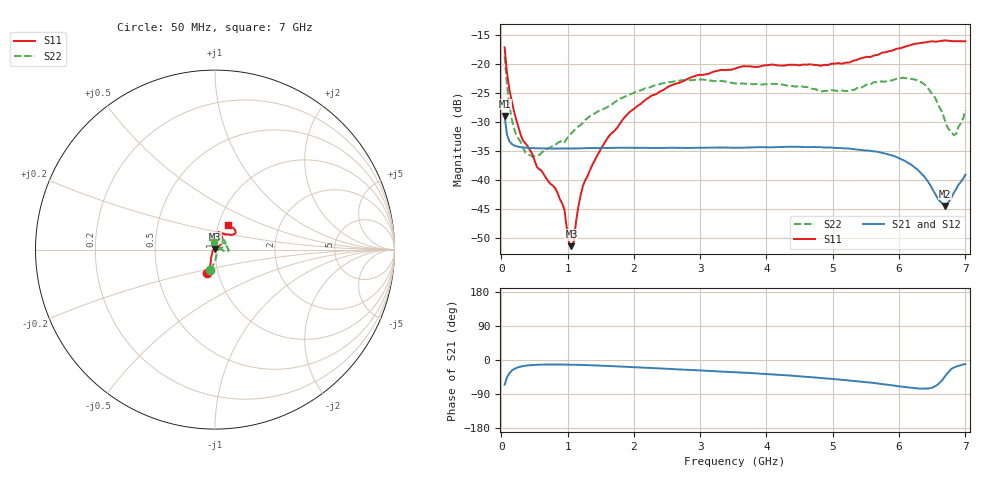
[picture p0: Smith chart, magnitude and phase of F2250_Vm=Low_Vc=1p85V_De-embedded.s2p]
! Integrated Device Technology
! Corporate Headquarters
! 6024 Silver Creek Valley Road
! San Jose, CA 95138  USA
! Phone:  1-408-284-8200
! Toll Free:  1-800-223-1366
! Webpage:  http://www.idt.com/
! Timing and RF Division
! 515 Groton Road, Suite 102
! Westford, MA 01886-6024
! Device:  F2250
! Description: Voltage Variable RF Attenuator
! Frequency:  50.0 -  6000.00 MHz
! Package:  3x3 mm Thin QFN Plastic Package: 16 pin
! Ports:  2 RF, 3 DC
!  Pin  1  = GND
!  Pin  2  = NC
!  Pin  3  = RF1  = Port 1
!  Pin  4  = NC
!  Pin  5  = GND
!  Pin  6  = GND
!  Pin  7  = GND
!  Pin  8  = GND
!  Pin  9  = NC
!  Pin 10  = RF2  = Port 2
!  Pin 11  = NC
!  Pin 12  = GND
!  Pin 13  = GND
!  Pin 14  = VCNTRL
!  Pin 15  = VDD
!  Pin 16  = VMODE
! Vcntrl:  1.850 Volts
! Vmode:  +0.000 Volts
! Vdd:  +3.30  Volts
! Current:  1.186 mA
! Data:  The device was measured on a the F2250 evaluation board which has
!  individual transmission lines to the RF pins.  Data was collected
!  using a calibrated network analyzer.  The evaluation board was
!  de-embedded using a TRL calibration technique.
!  The reference plane is the edge of the package pin.
! Misc:  SN 10
!  Action Tracker AT0258
! Date Measured:  2014-11-26
! Date:  2015-10-15  MJV
! Note:
!  Integrated Device Technology supplies this data as a sample of measured
!  data at the package pin for this product.  Your particular data for this
!  product may vary.
!  Data was taken at 25 degrees C.
!  Integrated Device Technology reserves the right to change this data at anytime.
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# GHz S dB R 50
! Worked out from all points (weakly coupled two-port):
!   201 points, 50 MHz to 7 GHz, reference 50 ohm
!   highest |S21| = -28.97 dB at 50 MHz (marker M1); lowest = -44.4 dB at 6.687 GHz (marker M2)
!   lowest |S11| = -51.3 dB at 1.058 GHz (marker M3), VSWR 1.01, Z = 49.9 + j0.236 ohm
!   |S11| at or under -10 dB: start of sweep to end of sweep
!   |S22| runs from -35.9 to -18.7 dB; largest |S21 - S12| = 5.1e-05
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0.05  -17.17 -108.4  -28.97 -65.3  -28.97 -65.3  -18.74 -102.7
0.08475  -21.44 -107.2  -32.13 -46.5  -32.13 -46.4  -23.53 -89.5
0.15425  -26.24 -116.2  -33.74 -28.7  -33.74 -28.7  -29.30 -78.5
0.29325  -32.23 -127.1  -34.33 -17.3  -34.33 -17.3  -33.49 -50.1
0.36275  -33.65 -138.4  -34.42 -15.1  -34.42 -15.1  -35.23 -33.0
0.57125  -38.08 -159.8  -34.52 -12.4  -34.52 -12.4  -35.69 -7.7
0.91875  -43.96 158.1  -34.57 -12.0  -34.56 -12.1  -33.20 4.6
0.9535  -45.11 170.1  -34.56 -12.1  -34.57 -12.1  -33.49 7.9
1.023  -50.85 143.3  -34.56 -12.3  -34.56 -12.3  -32.31 10.7
1.05775  -51.32 119.2  -34.56 -12.4  -34.56 -12.3  -31.93 11.7
1.0925  -50.66 85.0  -34.55 -12.5  -34.55 -12.5  -31.54 11.3
1.162  -44.52 53.9  -34.54 -12.8  -34.53 -12.7  -30.79 10.3
1.2315  -40.98 42.5  -34.51 -13.1  -34.51 -13.1  -30.13 9.9
1.6485  -32.08 41.4  -34.45 -16.0  -34.45 -16.0  -27.13 19.0
2.37825  -24.87 47.0  -34.44 -22.2  -34.44 -22.2  -23.56 29.1
3.525  -20.82 72.4  -34.42 -32.3  -34.42 -32.3  -23.37 56.8
4.7065  -20.19 72.3  -34.28 -45.8  -34.28 -45.8  -24.32 60.9
5.85325  -17.83 40.4  -35.61 -65.9  -35.61 -65.9  -22.86 5.4
6.3745  -16.34 41.3  -39.29 -75.6  -39.30 -75.6  -23.46 -9.2
6.68725  -16.00 48.7  -44.40 -44.3  -44.39 -43.9  -29.60 9.6
6.82625  -16.14 53.5  -42.14 -19.9  -42.11 -19.8  -32.27 50.4
7  -16.13 63.2  -39.04 -11.0  -39.00 -11.1  -27.96 97.9
